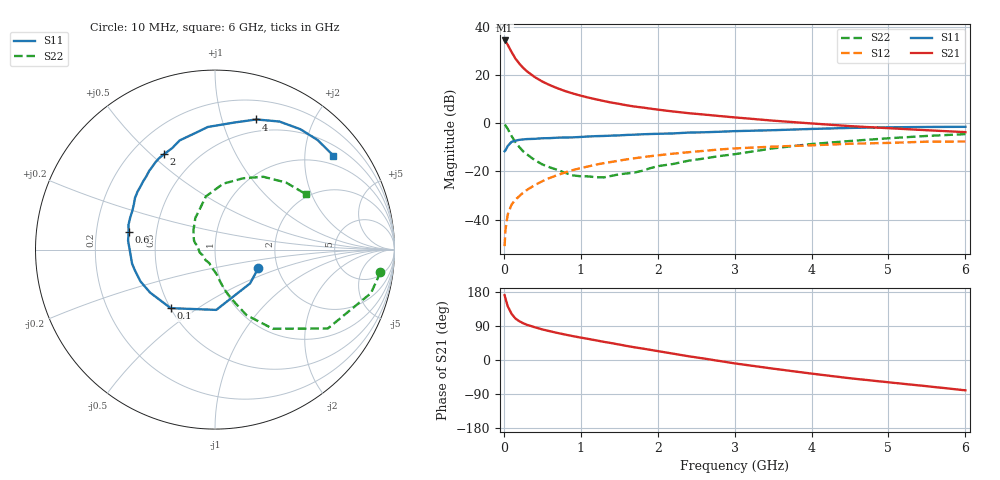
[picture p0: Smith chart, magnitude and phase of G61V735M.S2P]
! SIEMENS Small Signal Semiconductors
! BFG193
! Si NPN RF Bipolar Junction Transistor in SOT223
! VCE = 1.75 V  IC = 35 mA
! Common Emitter S-Parameters:  August  1996
# GHz  S  MA  R  50
!  f  S11  S21  S12  S22
! GHz  MAG  ANG  MAG  ANG  MAG  ANG  MAG  ANG
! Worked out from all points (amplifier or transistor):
!   36 points, 10 MHz to 6 GHz, reference 50 ohm
!   highest |S21| = 34.4 dB at 10 MHz (marker M1)
!   |S21| within 3 dB of that: start of sweep to 70.38 MHz
!   unconditionally stable (mu >= 1): 469.3 MHz to 2.638 GHz
!   at 250 MHz: K = 0.88, MSG = 26.0 dB, |S12| = -28.9 dB
!   at 1.4 GHz: K = 1.05, MAG = 10.9 dB, |S12| = -16.1 dB
!   at 6 GHz: K = 0.93, MSG = 2.0 dB, |S12| = -7.6 dB
!   S11 on the Smith chart (normalised r, x): 10 MHz: 1.58, -0.36; 100 MHz: 0.50, -0.39; 600 MHz: 0.34, +0.09; 2 GHz: 0.33, +0.55; 4 GHz: 0.38, +1.30; 6 GHz: 0.74, +2.68
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0.01  0.262 -23.6  52.3 171.1  0.0028 88.8  0.9303 -7.8
0.02  0.2715 -43.9  50.7 163.3  0.0059 83.0  0.9022 -15.6
0.05  0.336 -88.8  42.61 142.1  0.0126 69.0  0.7669 -35.0
0.1  0.4091 -127.1  30.19 122.0  0.0204 62.2  0.5455 -53.9
0.15  0.4338 -146.5  22.09 109.6  0.0258 60.8  0.4052 -64.3
0.2  0.4514 -156.9  17.38 102.5  0.0305 62.9  0.3218 -69.0
0.25  0.4599 -164.6  14.17 97.1  0.0359 62.8  0.2614 -73.6
0.3  0.4685 -170.2  11.99 92.9  0.0411 64.5  0.2262 -76.8
0.4  0.474 -178.9  9.119 86.6  0.0518 65.0  0.1723 -81.8
0.5  0.4869 174.1  7.334 80.7  0.0626 64.6  0.1396 -85.9
0.6  0.4907 168.6  6.159 75.9  0.0734 63.9  0.1211 -90.9
0.8  0.5053 159.1  4.631 67.0  0.0954 60.9  0.0931 -105.3
1.1  0.5307 147.1  3.399 55.5  0.1271 55.8  0.0787 -131.7
1.6  0.5715 130.0  2.352 37.0  0.1779 44.7  0.0906 -178.2
2  0.6026 118.1  1.917 23.6  0.2151 35.5  0.1283 156.0
2.2  0.6139 112.8  1.751 16.8  0.2333 30.8  0.1424 147.0
2.8  0.665 97.8  1.413 -2.5  0.285 16.5  0.2079 121.9
3.5  0.7163 81.3  1.131 -22.8  0.3269 -1.0  0.3008 99.7
4  0.7608 72.4  0.989 -35.9  0.3476 -10.8  0.37 82.9
4.5  0.7987 63.3  0.871 -48.2  0.3749 -20.8  0.4275 68.4
5.5  0.8364 46.8  0.715 -69.2  0.4138 -43.6  0.5442 43.4
6  0.842 38.5  0.653 -80.0  0.4163 -56.7  0.5937 31.3
